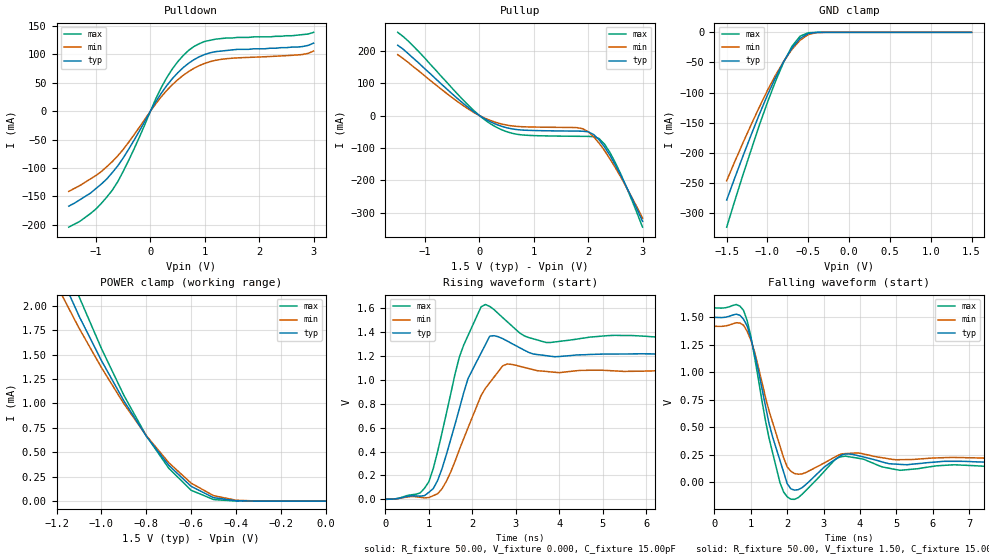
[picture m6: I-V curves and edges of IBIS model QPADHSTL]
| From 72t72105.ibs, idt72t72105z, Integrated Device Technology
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|   Model QPADHSTL
[Model]   QPADHSTL
Model_type   3-state
Polarity   Non-Inverting
Enable   Active-High
Vmeas =  0.750V
C_comp   3.00pF   NA   NA
[Temperature Range]   25.00   85.00   -40.00
[Voltage Range]   1.50V   1.40V   1.60V
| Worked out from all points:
|   slope of the pulldown table from 0 to 0.225 V, typ, clamps not added: 6.42 ohm
|   slope of the pullup table from 0 to 0.225 V, typ, clamps not added: 10.7 ohm
|   GND clamp passes 1 mA (typ) near -0.45 V on its own axis
|   POWER clamp passes 1 mA (typ) near -0.89 V on its own axis
|   rising waveform, R_fixture 50.00, V_fixture 0.000, C_fixture 15.00pF: 20-80 % time 580ps typ, 707ps min, 518ps max; typ from 0 V to 1.22 V
|   falling waveform, R_fixture 50.00, V_fixture 1.50, C_fixture 15.00pF: 20-80 % time 518ps typ, 570ps min, 464ps max; typ from 1.5 V to 0.183 V
[Pulldown]
| voltage   I(typ)   I(min)   I(max)
-1.5V     -167mA     -141mA     -204mA
-1.3V     -156mA     -131mA     -194mA
-1V       -136mA     -113mA     -172mA
-700mV    -108mA     -88.57mA   -139mA
-400mV    -66.98mA   -54.66mA   -86.64mA
200mV     31.71mA    25.58mA    41.77mA
400mV     57.04mA    46.47mA    74.01mA
700mV     84.35mA    69.78mA    107mA
1V        100mA      84.36mA    123mA
1.2V      105mA      89.75mA    127mA
2.7V      113mA      99.15mA    134mA
3V        120mA      106mA      139mA
[Pullup]
| voltage   I(typ)   I(min)   I(max)
-1.5V     217mA      188mA      257mA
-1.1V     160mA      136mA      195mA
-300mV    37.97mA    30.98mA    48.44mA
0V        0A         -10pA      30pA
300mV     -26.66mA   -21.07mA   -35.09mA
800mV     -45.1mA    -34.74mA   -60.27mA
1.9V      -48.49mA   -40.89mA   -64.4mA
2.1V      -58.61mA   -65.59mA   -65.33mA
2.2V      -74.81mA   -85.32mA   -71.21mA
2.3V      -96.98mA   -108mA     -88.2mA
2.5V      -153mA     -161mA     -146mA
3V        -327mA     -317mA     -345mA
[GND_clamp]
| voltage   I(typ)   I(min)   I(max)
-1.5V     -278mA     -246mA     -323mA
-1.3V     -205mA     -183mA     -236mA
-1.1V     -136mA     -124mA     -154mA
-1V       -104mA     -96.2mA    -116mA
-900mV    -74.56mA   -70.77mA   -80.61mA
-800mV    -48.24mA   -47.87mA   -49.04mA
-700mV    -26.16mA   -28.23mA   -23.28mA
-600mV    -10.07mA   -12.98mA   -6.406mA
-500mV    -2.002mA   -3.724mA   -655uA
-400mV    -177uA     -538uA     -28.11uA
1.5V      15.11nA    22.17nA    15nA
[POWER_clamp]
| voltage   I(typ)   I(min)   I(max)
-1.5V     8.542mA    5.787mA    13.11mA
-1.2V     2.409mA    2.216mA    2.73mA
-1.1V     1.896mA    1.773mA    2.096mA
-1V       1.44mA     1.368mA    1.563mA
-900mV    1.027mA    998uA      1.084mA
-800mV    665uA      671uA      669uA
-700mV    367uA      394uA      337uA
-600mV    151uA      184uA      111uA
-500mV    35.56uA    56.06uA    16.17uA
-400mV    4.035uA    9.223uA    1.078uA
0V        15.11nA    18.77nA    16nA
[Ramp]
| variable   typ   min   max
dV/dt_r   0.74/0.49n   0.65/0.65n   0.83/0.38n
dV/dt_f   0.80/0.40n   0.73/0.47n   0.88/0.31n
R_load = 50.00
[Rising Waveform]
R_fixture = 50.00
V_fixture = 0.000
C_fixture = 15.00pF
R_dut = 0.75
L_dut = 8.10nH
C_dut = 0.53pF
| time   V(typ)   V(min)   V(max)
0s        0V         0V         0V
1ns       59.11mV    15.18mV    148mV
1.3ns     255mV      87.23mV    555mV
1.7ns     757mV      415mV      1.19V
1.9ns     1.01V      598mV      1.37V
2.3ns     1.294V     929mV      1.63V
2.4ns     1.365V     976mV      1.614V
2.8ns     1.325V     1.132V     1.487V
3.7ns     1.202V     1.07V      1.312V
9.9ns     1.215V     1.075V     1.359V
[Falling Waveform]
R_fixture = 50.00
V_fixture = 1.50
C_fixture = 15.00pF
R_dut = 0.75
L_dut = 8.10nH
C_dut = 0.53pF
| time   V(typ)   V(min)   V(max)
0s        1.5V       1.419V     1.586V
800ps     1.483V     1.429V     1.564V
1.1ns     1.171V     1.189V     1.143V
1.4ns     698mV      777mV      564mV
1.8ns     199mV      330mV      -3.805mV
2.1ns     -60.67mV   99.63mV    -155mV
2.4ns     -51.48mV   75.18mV    -113mV
3.6ns     257mV      260mV      237mV
5.1ns     162mV      205mV      108mV
9.9ns     183mV      220mV      145mV
